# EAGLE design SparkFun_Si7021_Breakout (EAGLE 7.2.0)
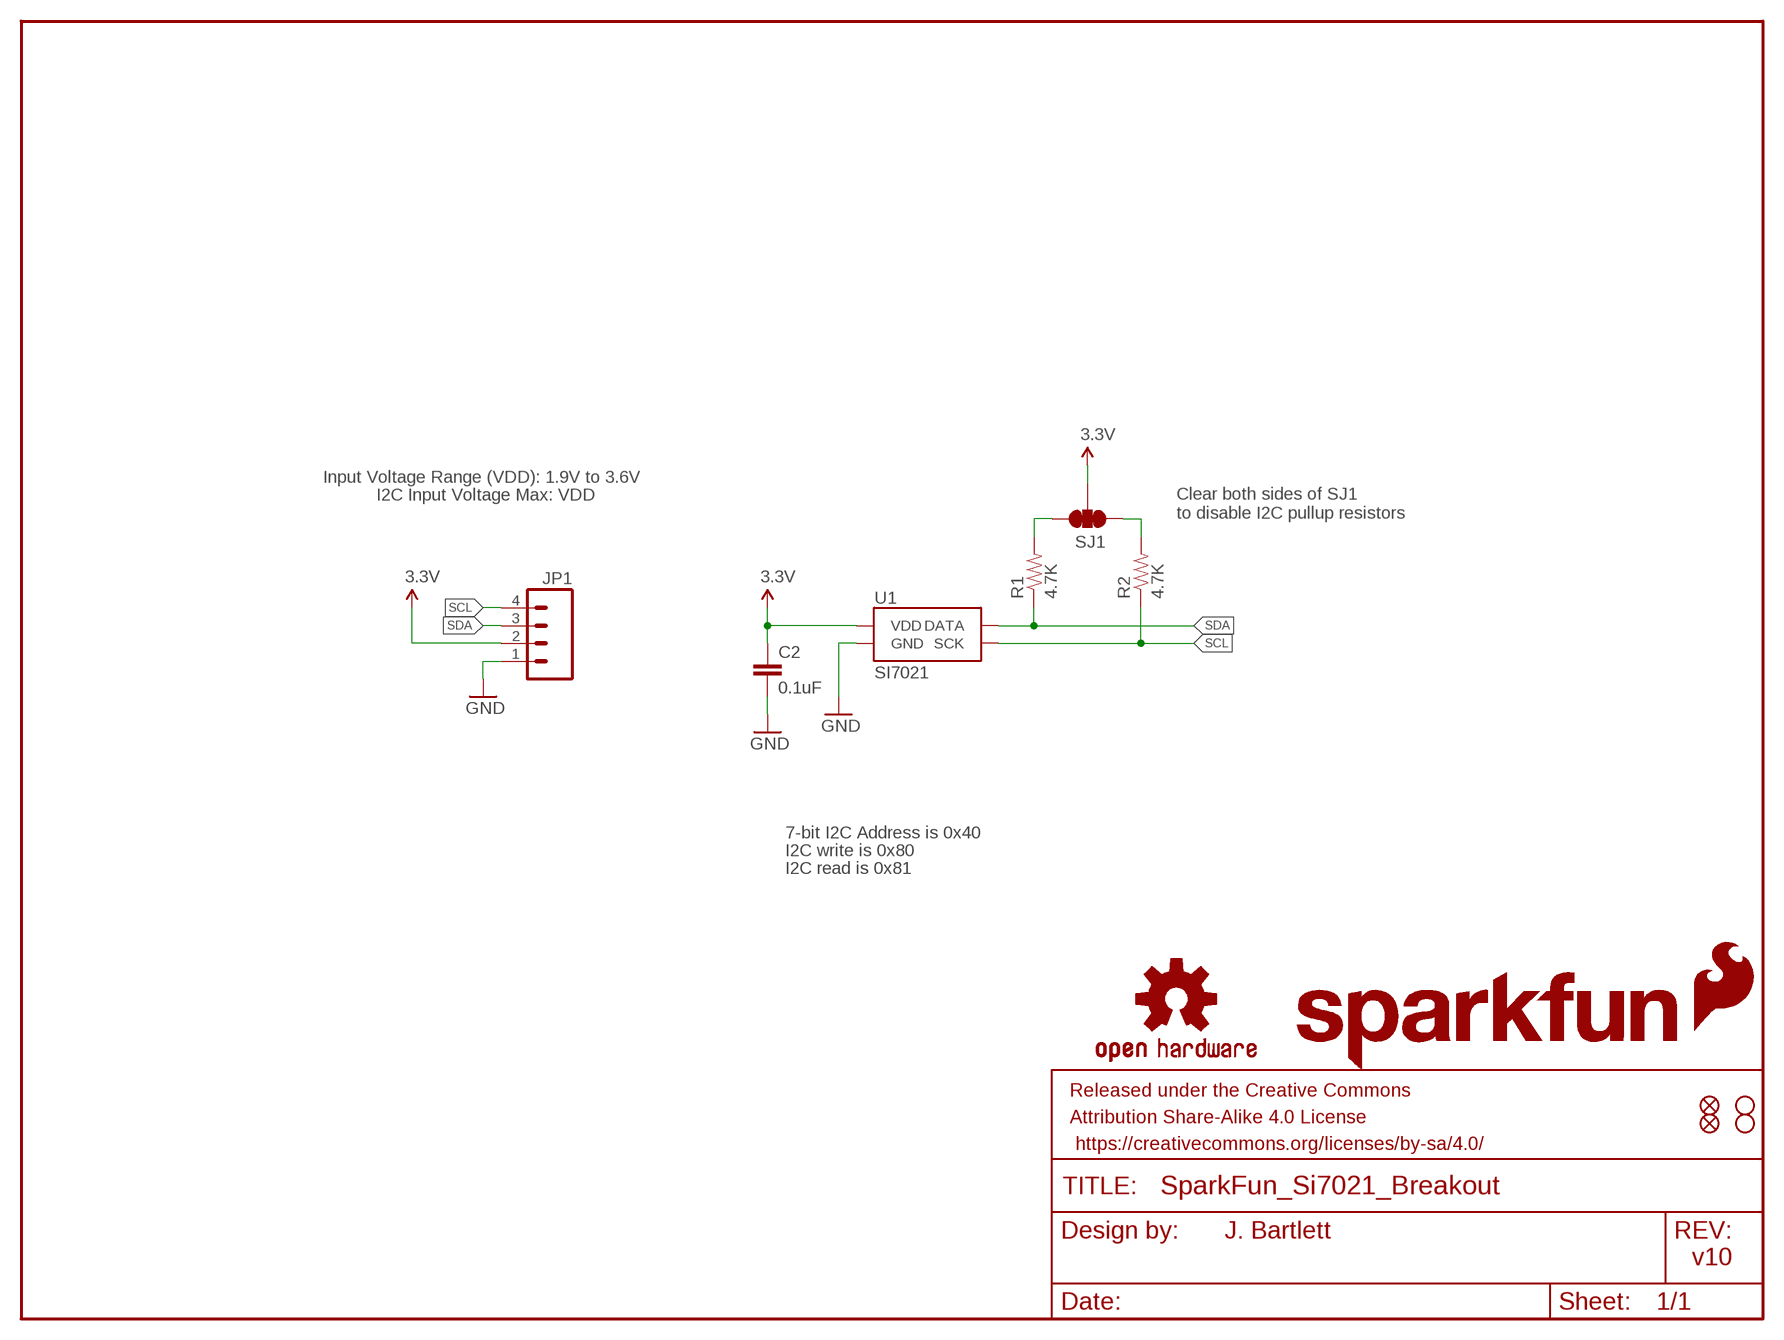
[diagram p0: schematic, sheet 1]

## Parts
C2  0.1uF  0.1UF-25V(+80/-20%)(0603)  [0603-CAP]
FRAME2  FRAME-LETTER  [CREATIVE_COMMONS]
JP1  M04PTH  [1X04]
JP3  FIDUCIALUFIDUCIAL  [MICRO-FIDUCIAL]
JP4  FIDUCIALUFIDUCIAL  [MICRO-FIDUCIAL]
LOGO2  OSHW-LOGOS  [OSHW-LOGO-S]
LOGO3  SFE_LOGO_FLAME.1_INCH  [SFE_LOGO_FLAME_.1]
LOGO4  SFE_LOGO_NAME.1_INCH  [SFE_LOGO_NAME_.1]
R1  4.7K  4.7KOHM-1/10W-1%(0603)  [0603-RES]
R2  4.7K  4.7KOHM-1/10W-1%(0603)  [0603-RES]
SJ1  SOLDERJUMPER_2WAYPASTE1&2&3  [SJ_3_PASTE1&2&3]
STANDOFF1  STAND-OFF  [STAND-OFF]
STANDOFF2  STAND-OFF  [STAND-OFF]
U1  SI7021  [SI7021]

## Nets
3.3V: C2.1 JP1.2 SJ1.2 U1.VDD
GND: C2.2 JP1.1 U1.GND
N$1: R1.2 SJ1.3
N$2: R2.2 SJ1.1
SCL: JP1.4 R2.1 U1.SCK
SDA: JP1.3 R1.1 U1.DATA

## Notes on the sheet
- Input Voltage Range (VDD): 1.9V to 3.6V
- I2C Input Voltage Max: VDD
- Clear both sides of SJ1
  to disable I2C pullup resistors
- 7-bit I2C Address is 0x40
- I2C write is 0x80
- I2C read is 0x81
- J. Bartlett
- v10

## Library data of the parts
C2 = SparkFun-Capacitors:0.1UF-25V(+80/-20%)(0603): CAP-00810; PROD_ID: CAP-00810
FRAME2 = SparkFun-Aesthetics:FRAME-LETTER: Schematic Frame
JP1 = SparkFun-Connectors:M04: Header 4 Standard 4-pin 0.1" header. Use with straight break away headers (SKU : PRT-00116), right angle break away headers (PRT-00553), swiss pins (PRT-00743), machine pins (PRT-00117), and female headers (PRT-00115). Molex polarized connector foot print use with SKU : PRT-08231 with associated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
JP3 JP4 = SparkFun-Aesthetics:FIDUCIAL: Fiducial Alignment Points
LOGO2 = SparkFun-Aesthetics:OSHW-LOGO: Open Source Hardware Logo This logo indicates the piece of hardware it is found on incorporates a OSHW license and/or adheres to the definition of open source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
LOGO3 = SparkFun-Aesthetics:SFE_LOGO_FLAME: SFE Logo, flame only
LOGO4 = SparkFun-Aesthetics:SFE_LOGO_NAME: SFE Logo, name only
R1 R2 = SparkFun-Resistors:4.7KOHM-1/10W-1%(0603): RES-07857; PROD_ID: RES-07857
SJ1 = mike-temp:SOLDERJUMPER_2WAY: Solder Jumper 2 way solder jumper
STANDOFF1 STANDOFF2 = SparkFun-Electromechanical:STAND-OFF: #4 Stand Off
U1 = SparkFun-Sensors:SI7021: The Si7021 is an I2C Humidity and Temperature Sensor; PROD_ID: IC-13093

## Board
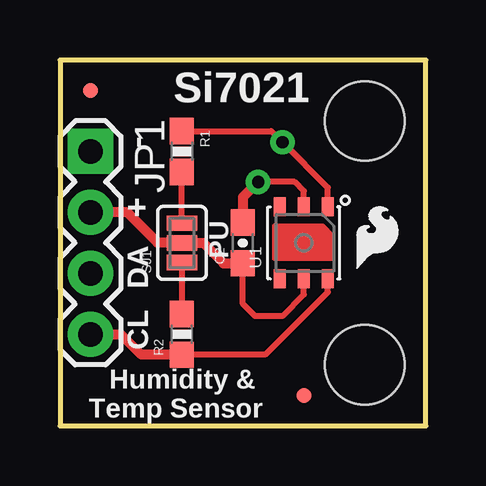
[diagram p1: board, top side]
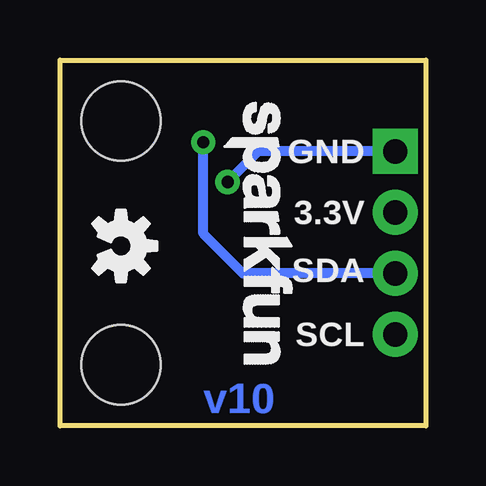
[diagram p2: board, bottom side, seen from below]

Size 15.24 x 15.24 mm. Coordinates in mm from the lower left corner, seen from the top.
Outline: 15.24,0 15.24,15.24 0,15.24 0,0 15.24,0
Copper layers (1*16): Top 0.035mm / dielectric 1.5mm / Bottom 0.035mm
Design rules "SparkFun": minimum track width 8mil, minimum drill 20mil, track to track 8mil, track to pad 8mil, pad to pad 8mil, via to via 8mil, smd to smd 8mil, copper to edge 10mil, drill to drill 8mil, minimum pad ring 12mil, minimum via ring 10mil, stop-mask expansion 4mil, vias tented up to drill 25mil, thermal gap 10mil

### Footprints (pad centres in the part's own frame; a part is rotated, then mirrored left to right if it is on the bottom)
0603-CAP = smd 1.1 x 1: 1 -0.85,0; 2 0.85,0
1X04 = drill 1.016 pad 1.88 square: 1 0,0 | drill 1.016 pad 1.88: 2 2.54,0; 3 5.08,0; 4 7.62,0
MICRO-FIDUCIAL = smd 0.635 x 0.635: 1 0,0
0603-RES = smd 1.1 x 1: 1 -0.85,0; 2 0.85,0
SJ_3_PASTE1&2&3 = smd 0.635 x 1.27: 1 -0.813,0; 2 0,0; 3 0.813,0
STAND-OFF = hole 3.302: 0,0
SI7021 = smd 0.8 x 0.5: DATA 1.5,-1; GND 1.5,0; NC@3 1.5,1; NC@4 -1.5,1; SCK -1.5,-1; VDD -1.5,0

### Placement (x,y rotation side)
C2  7.62,7.62 90 top
FRAME2  not placed on the board
JP1  1.27,11.43 270 top
JP3  10.16,1.27 90 top
JP4  1.27,13.97 90 top
LOGO2  12.7,7.49 270 bottom
LOGO3  12.06,6.22 0 top
LOGO4  8.89,13.97 270 bottom
R1  5.08,11.43 270 top
R2  5.08,3.81 90 top
SJ1  5.08,7.62 90 top
STANDOFF1  12.7,12.7 90 top
STANDOFF2  12.7,2.54 90 top
U1  10.16,7.62 90 top

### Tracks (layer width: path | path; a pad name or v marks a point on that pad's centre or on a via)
3.3V
  Top 0.254: U1.VDD 10.16,5.46 9.27,4.57 8.13,4.57 7.62,5.08 C2.1
  Top 0.406: JP1.2 2.79,8.89 4.06,7.62 SJ1.2 5.97,7.62 6.82,6.77 C2.1
GND  (via drill 0.51)
  Top 0.254: U1.GND 10.16,9.78 9.78,10.16 v8.26,10.16
  Top 0.406: v8.26,10.16 7.62,9.53 C2.2
  Bottom 0.406: JP1.1 6.99,11.43 v8.26,10.16
N$1
  Top 0.254: SJ1.3 R1.2
N$2
  Top 0.254: SJ1.1 R2.2
SCL
  Top 0.254: U1.SCK 11.16,5.57 8.55,2.96 R2.1
  Top 0.406: JP1.4 2.54,3.81 3.39,2.96 R2.1
SDA  (via drill 0.51)
  Top 0.254: U1.DATA 11.16,9.92 v9.27,11.81 8.8,12.28 R1.1
  Bottom 0.406: JP1.3 7.62,6.35 9.27,8 v9.27,11.81

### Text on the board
Bottom: v10
tPlace: Si7021 | - | + | PU | DA | CL | Humidity & / Temp Sensor
bPlace: GND | 3.3V | SDA | SCL
tDocu: J. Bartlett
